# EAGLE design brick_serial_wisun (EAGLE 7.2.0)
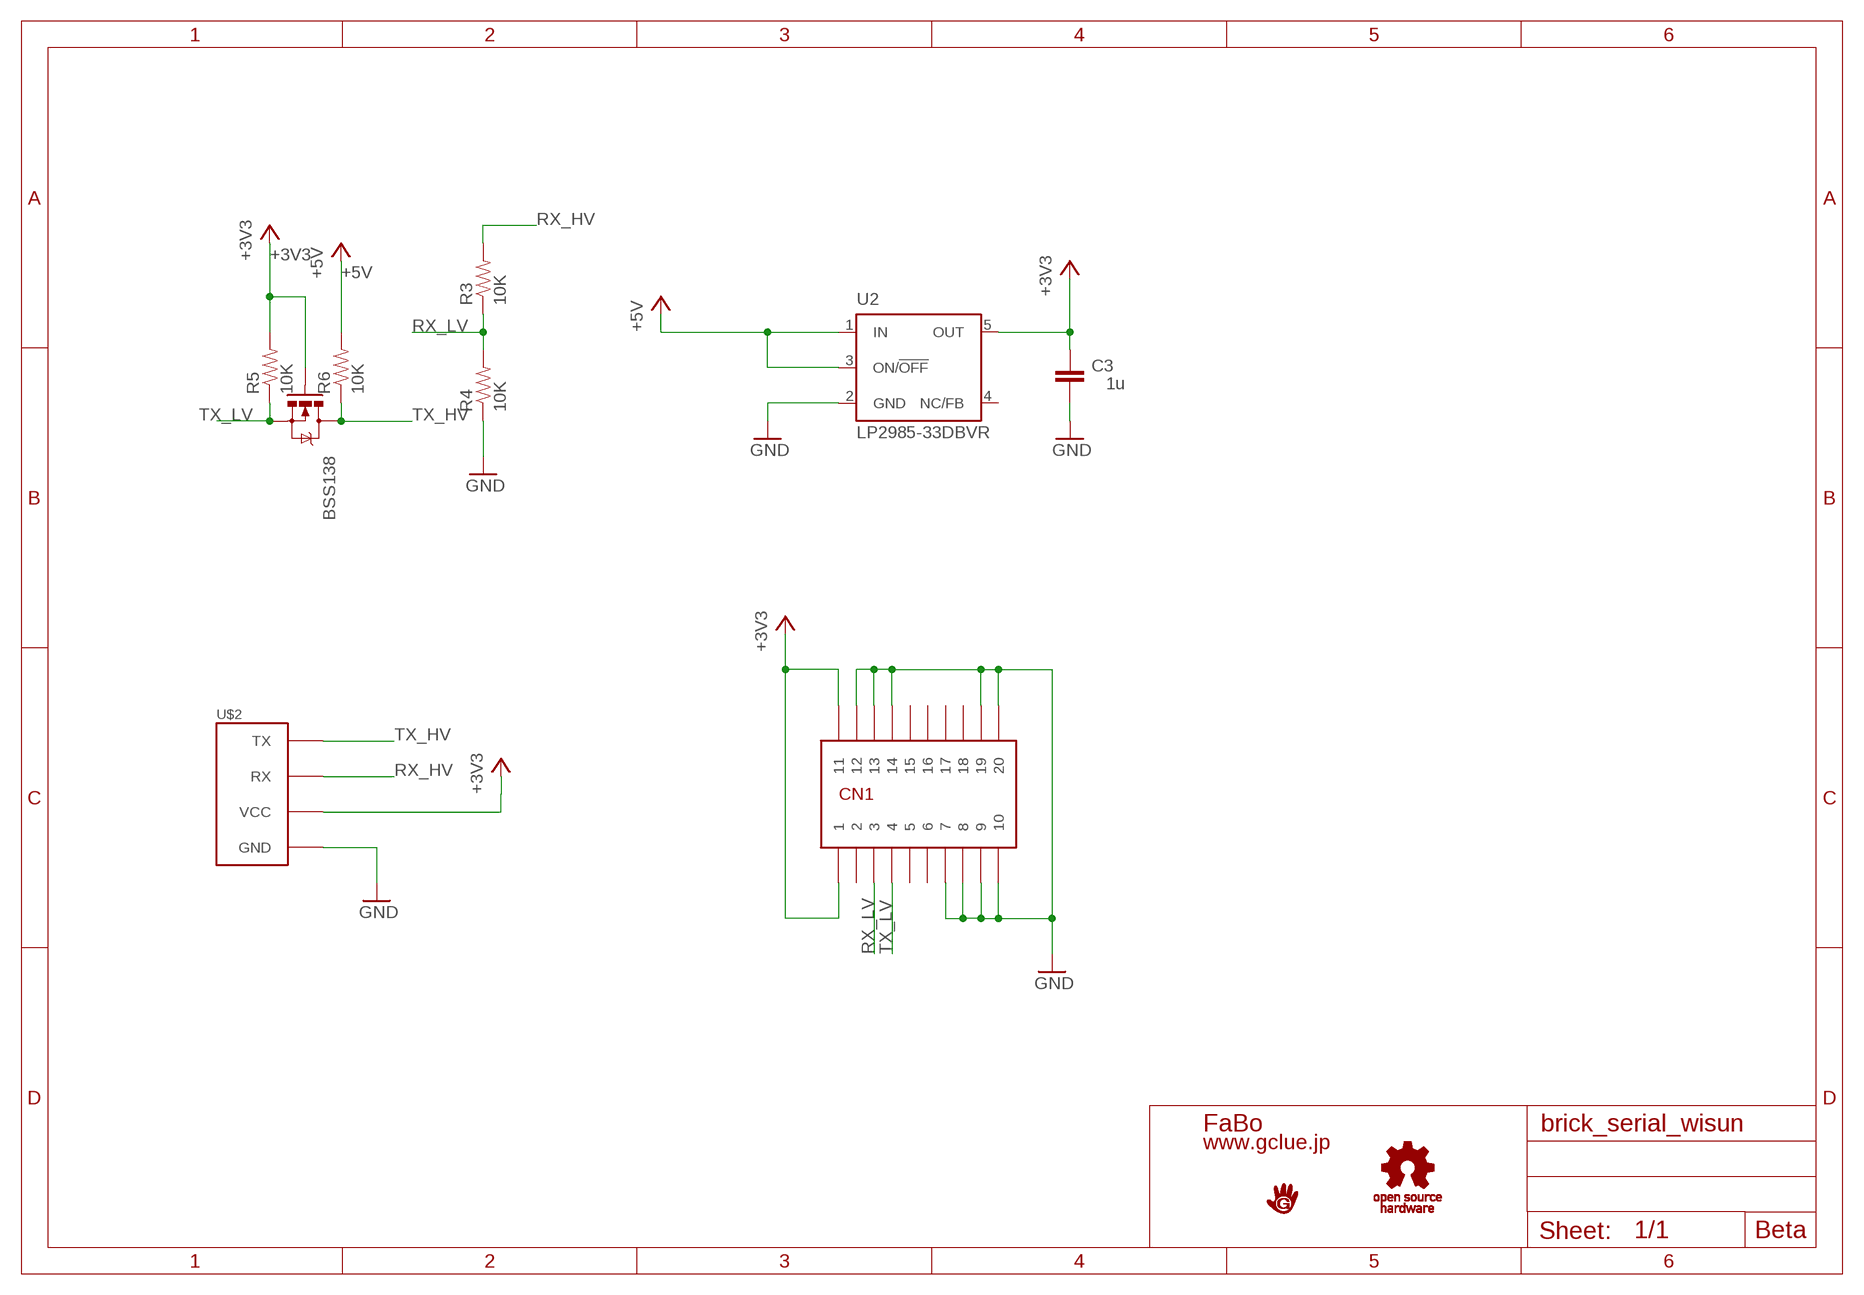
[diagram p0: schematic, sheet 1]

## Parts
BSS138  MOSFET-NCHANNELSMD  [SOT23-3]
C3  1u  C-EU0603-RND  [C0603-ROUND]
CN1  JST-20P3.0-JMCS  [JST-20P3.0-JMCS]
R3  10K  RESISTOR0603-RES  [0603-RES]
R4  10K  RESISTOR0603-RES  [0603-RES]
R5  10K  RESISTOR0603-RES  [0603-RES]
R6  10K  RESISTOR0603-RES  [0603-RES]
U2  LP2985-33DBVR  LP2985-XXDBVR33  [SOT23-DBV]
U$1  LOGO_GCLUE-M  [LOGO_GCLUE_M]
U$2  BRICK_SERIAL  [BRICK_SERIAL]
U$4  LOGO_OSHW_T-M  [LOGO_OSHW_T_M]

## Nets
+3V3 [PWR]: BSS138.1(G) C3.2 CN1.10 CN1.20 R5.2 U2.5(OUT) U$2.VCC
+5V [PWR]: R6.2 U2.1(IN) U2.3(ON/!OFF)
GND [PWR]: C3.1 CN1.1 CN1.2 CN1.3 CN1.4 CN1.11 CN1.12 CN1.17 CN1.18 CN1.19 R4.1 U2.2(GND) U$2.GND
RX_HV: R3.2 U$2.RX
RX_LV: CN1.8 R3.1 R4.2
TX_HV: BSS138.3(D) R6.1 U$2.TX
TX_LV: BSS138.2(S) CN1.7 R5.1
Unconnected: CN1.5 CN1.6 CN1.9 CN1.13 CN1.14 CN1.15 CN1.16 U2.4(NC/FB)

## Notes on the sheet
- Beta

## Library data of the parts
BSS138 = SparkFun:MOSFET-NCHANNEL
C3 = SmartPrj:C-EU: CAPACITOR, European symbol
CN1 = gclueParts:JST-20P3.0-JMCS
R3-R6 = SparkFun:RESISTOR: Resistor
U2 = SmartPrj:LP2985-XXDBVR: ULTRALOW-POWER 50-mA LOW-DROPOUT LINEAR REGULATORS 50-mA Low-Dropout Regulator Source: http://focus.ti.com/lit/ds/symlink/tps77001.pdf
U$1 = gclue:LOGO_GCLUE
U$2 = gclue:BRICK_SERIAL: FaBo Brick 4pin(SERIAL)
U$4 = gclue:LOGO_OSHW_T

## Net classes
1 PWR: width 0.254 mm

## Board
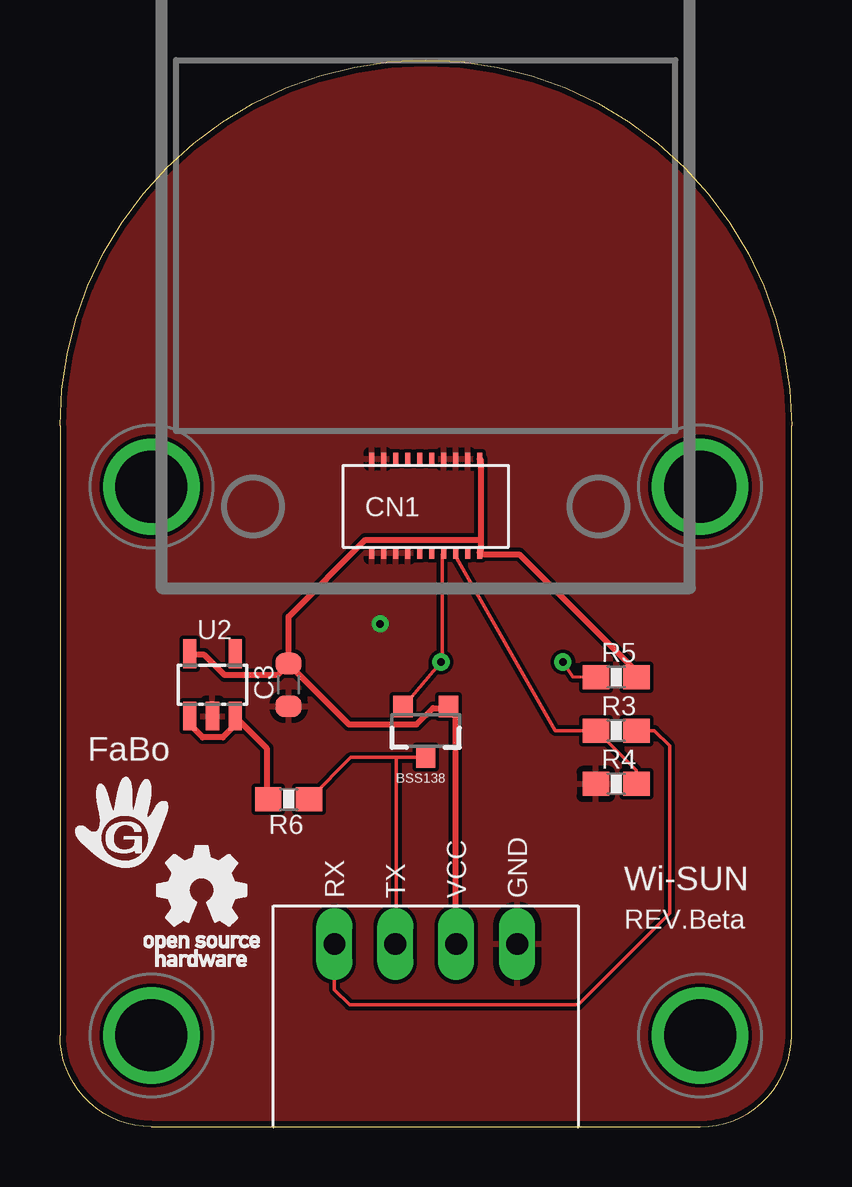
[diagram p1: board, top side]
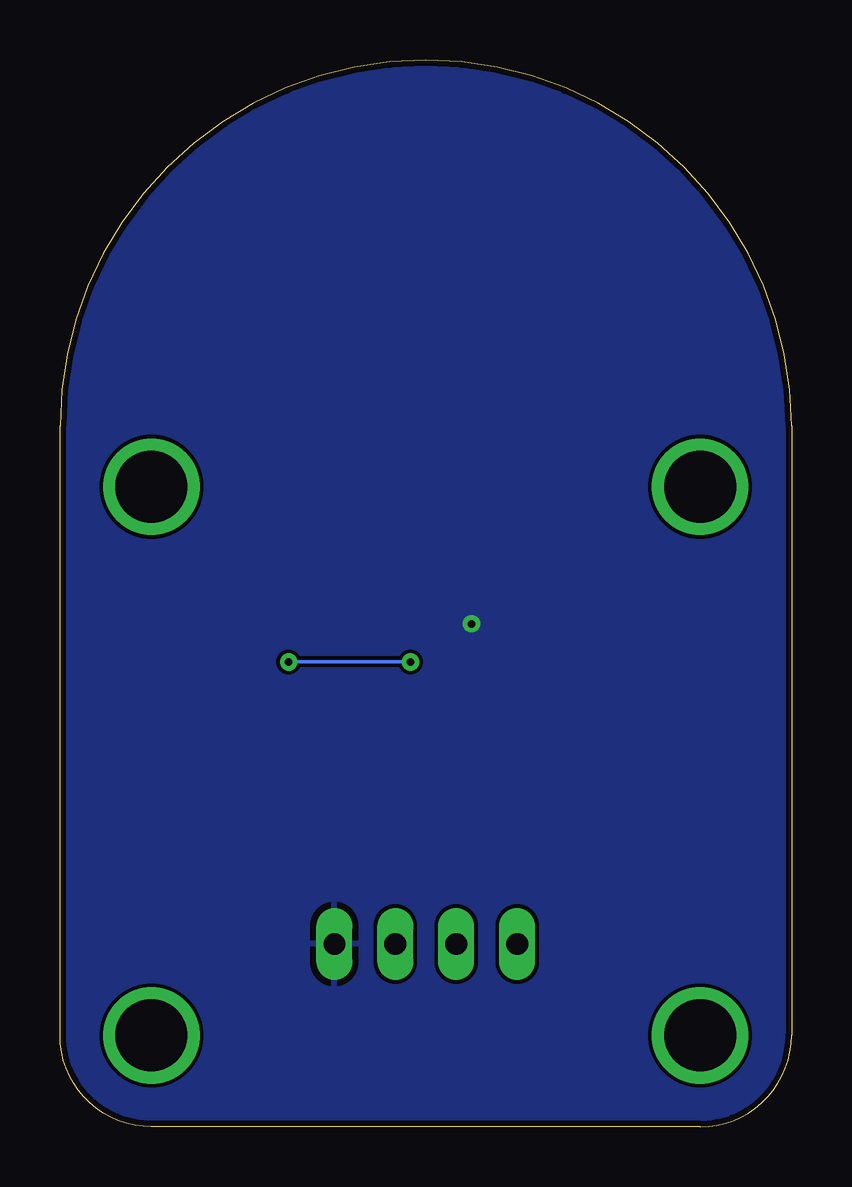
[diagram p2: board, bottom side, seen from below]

Size 30.48 x 44.45 mm. Coordinates in mm from the lower left corner, seen from the top.
Copper layers (1*16): Top 0.035mm / dielectric 1.5mm / Bottom 0.035mm
Design rules "DFRobot_Eagle_Rule_v0.4": minimum track width 6mil, minimum drill 12mil, track to track 6mil, track to pad 6mil, pad to pad 6mil, via to via 6mil, smd to smd 0mil, copper to edge 10mil, drill to drill 10mil, minimum pad ring 12mil, minimum via ring 8mil, stop-mask expansion 2mil, vias tented up to drill 25mil, thermal gap 10mil

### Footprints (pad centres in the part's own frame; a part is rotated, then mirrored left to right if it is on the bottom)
SOT23-3 = smd 0.8 x 0.9: 1 -0.95,-1; 2 0.95,-1; 3 0,1.1
C0603-ROUND = smd 0.898 x 1.1: 1 -0.889,0; 2 0.889,0
JST-20P3.0-JMCS = smd 0.2 x 0.5: 1 -2.252,-1.924; 2 -1.752,-1.924; 3 -1.252,-1.924; 4 -0.752,-1.924; 5 -0.252,-1.924; 6 0.248,-1.924; 7 0.748,-1.924; 8 1.248,-1.924; 9 1.748,-1.924; 10 2.248,-1.924; 11 -2.252,1.976; 12 -1.752,1.976; 13 -1.252,1.976; 14 -0.752,1.976; 15 -0.252,1.976; 16 0.248,1.976; 17 0.748,1.976; 18 1.248,1.976; 19 1.748,1.976; 20 2.248,1.976
0603-RES = smd 1.1 x 1: 1 -0.85,0; 2 0.85,0
SOT23-DBV = smd 0.55 x 1.2: 1 -0.95,-1.3; 2 0,-1.3; 3 0.95,-1.3; 4 0.95,1.3; 5 -0.95,1.3
BRICK_SERIAL = drill 0.9 long: GND 3.81,-11.43; RX -3.81,-11.43; TX -1.27,-11.43; VCC 1.27,-11.43 | drill 3 pad 3.81: P$5 -11.43,7.62; P$6 11.43,7.62; P$7 -11.43,-15.24; P$8 11.43,-15.24

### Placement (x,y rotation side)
BSS138  15.24,16.51 180 top
C3  9.53,18.41 90 top
CN1  15.24,25.85 0 top
R3  23.18,16.51 0 top
R4  23.18,14.29 0 top
R5  23.18,18.73 0 top
R6  9.53,13.65 180 top
U2  6.35,18.41 0 top
U$1  2.54,12.7 0 top
U$2  15.24,19.05 0 top
U$4  6.03,9.21 0 top

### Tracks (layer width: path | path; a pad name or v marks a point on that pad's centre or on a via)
+3V3
  Top 0.254: 17.53,24.46 17.53,27.81 CN1.20 | 17.53,24.46 17.53,23.93 | 17.53,23.93 CN1.10 | R5.2 24,18.75 24,18.97 19.13,23.85 17.6,23.85 17.53,23.93 | C3.2 9.53,19.28 12.04,16.76 14.86,16.76 15.54,17.45 16.15,17.45 BSS138.1 16.23,17.37 16.46,17.14 16.46,7.62 U$2.VCC | U2.5 5.41,19.66 6.02,19.66 6.86,18.82 9.07,18.82 9.45,19.2 C3.2 | 17.53,24.46 12.72,24.46 9.53,21.26 C3.2
+5V
  Top 0.254: R6.2 8.61,13.72 8.61,15.77 7.32,17.07 U2.3 7.39,16.84 6.78,16.23 5.94,16.23 5.41,16.76 5.41,17.07 U2.1
GND  (via drill 0.3)
  other vias: 13.34,20.95
  pour Bottom: -0.64,-0.64 31.11,-0.64 31.11,45.09 -0.64,45.09
  pour Top: -0.64,-0.64 31.11,-0.64 31.11,45.09 -0.64,45.09
RX_HV
  Top 0.152: R3.2 24.77,16.51 25.4,15.88 25.4,8.89 21.59,5.08 12.06,5.08 11.43,5.71 U$2.RX
RX_LV
  Top 0.152: CN1.8 16.54,23.85 16.54,23.7 20.64,16.51 R3.1 22.4,16.46 24,14.86 24,14.33 R4.2
TX_HV
  Top 0.152: 14.02,15.39 12.12,15.39 10.44,13.72 R6.1 | 14.02,15.39 15.24,15.39 BSS138.3 | 14.02,15.39 14.02,7.62 U$2.TX
TX_LV  (via drill 0.3)
  Top 0.152: CN1.7 15.93,23.85 15.93,19.44 v15.88,19.37 14.33,17.53 BSS138.2 | v20.95,19.37 21.37,18.75 R5.1
  Bottom 0.152: v15.88,19.37 v20.95,19.37

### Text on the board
tPlace: FaBo | Wi-SUN | REV.Beta

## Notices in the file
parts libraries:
SparkFun: Licensing: CC v3.0 Share-Alike You are welcome to use this library for commercial purposes.
